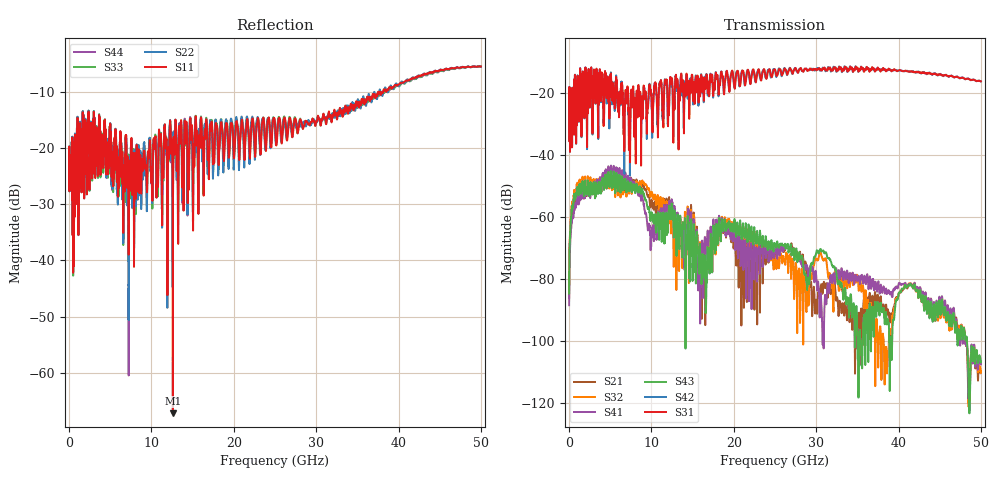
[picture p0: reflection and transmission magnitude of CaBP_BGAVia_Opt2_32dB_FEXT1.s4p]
!* Samtec Inc. NovaRay Examax Flyover System  *
!*  REV DATE  = 08/08/18  *
!*  TYPE  = TOUCHSTONE  *
!*  PORTS  = 4 port  *
!*  UNITS  = GHz  *
!*  DATA RANGE = DC  to 50 GHz; 10 MHz Step  *
!*  PARAMETER  = S  *
!*  FORMAT  = Real-Imaginary  *
!*  REFERENCE  = 50 ohms  *
!*  SOURCE  = HFSS  *
!*  VALIDATED  = No  *
!*  MANUFACTURER = SAMTEC  *
!*  INTERCONNECT = NVAx to EBCx to EBCx to NVAx  *
!*  [Full Channel NVAx to EBCx to EBCx to NVAx  with PCB Trace and BGA Via]  *
!*  BOUNDARY A  = Silicon BGA Ball Pad  *
!*  BOUNDARY B  = Silicon BGA Ball Pad  *
!*  NVAx (end a) ->>- (end b) NVAx  *
!*  Port 01 ->>- Port 02  *
!*  Port 03 ->>- Port 04  *
!***************************** CHANNEL MODEL ******************************************
# GHz S RI R 50
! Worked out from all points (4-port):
!   5000 points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, 10 MHz to 50 GHz, reference 50 ohm
!   strongest paths, dB at 10 MHz, 12.51 GHz, 25.01 GHz, 37.51 GHz, 50 GHz:
!     S31: -23.1, -15.2, -12.2, -11.7, -16.1
!     S42: -23.1, -16.0, -12.7, -12.0, -16.1
!     S43: -84.7, -58.0, -68.9, -88.2, -106.7
!     S41: -88.5, -55.8, -70.4, -81.6, -107.0
!     S32: -83.4, -60.7, -72.0, -106.0, -109.9
!     S21: -86.1, -58.2, -69.9, -85.7, -109.7
!   lowest |S11| = -67.2 dB at 12.6 GHz (marker M1), VSWR 1.00, Z = 50 + j0.0147 ohm
!   |S11| at or under -10 dB: start of sweep to 37.74 GHz; 37.74 GHz to 38.13 GHz (385.5 MHz wide, 1.02 % of centre); 38.51568 GHz to 38.54961 GHz (33.93 MHz wide, 0.0881 % of centre)
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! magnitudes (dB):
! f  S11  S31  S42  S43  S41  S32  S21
! 10 MHz  -21.6  -23.1  -23.1  -84.7  -88.5  -83.4  -86.1
! 790 MHz  -19.6  -17.6  -17.6  -53.5  -56.7  -52.3  -54.9
! 4.62 GHz  -20.5  -15.7  -16.1  -48.5  -47.2  -48.4  -48.1
! 12.6 GHz  -67.2  -21.8  -25.2  -60.0  -56.5  -63.8  -59.6
! 15.83 GHz  -18.3  -15.4  -15.3  -75.0  -70.5  -70.2  -68.9
! 18.35 GHz  -17.2  -16.4  -15.7  -65.4  -65.1  -64.5  -65.9
! 50 GHz  -5.5  -16.1  -16.1  -106.7  -107.0  -109.9  -109.7
